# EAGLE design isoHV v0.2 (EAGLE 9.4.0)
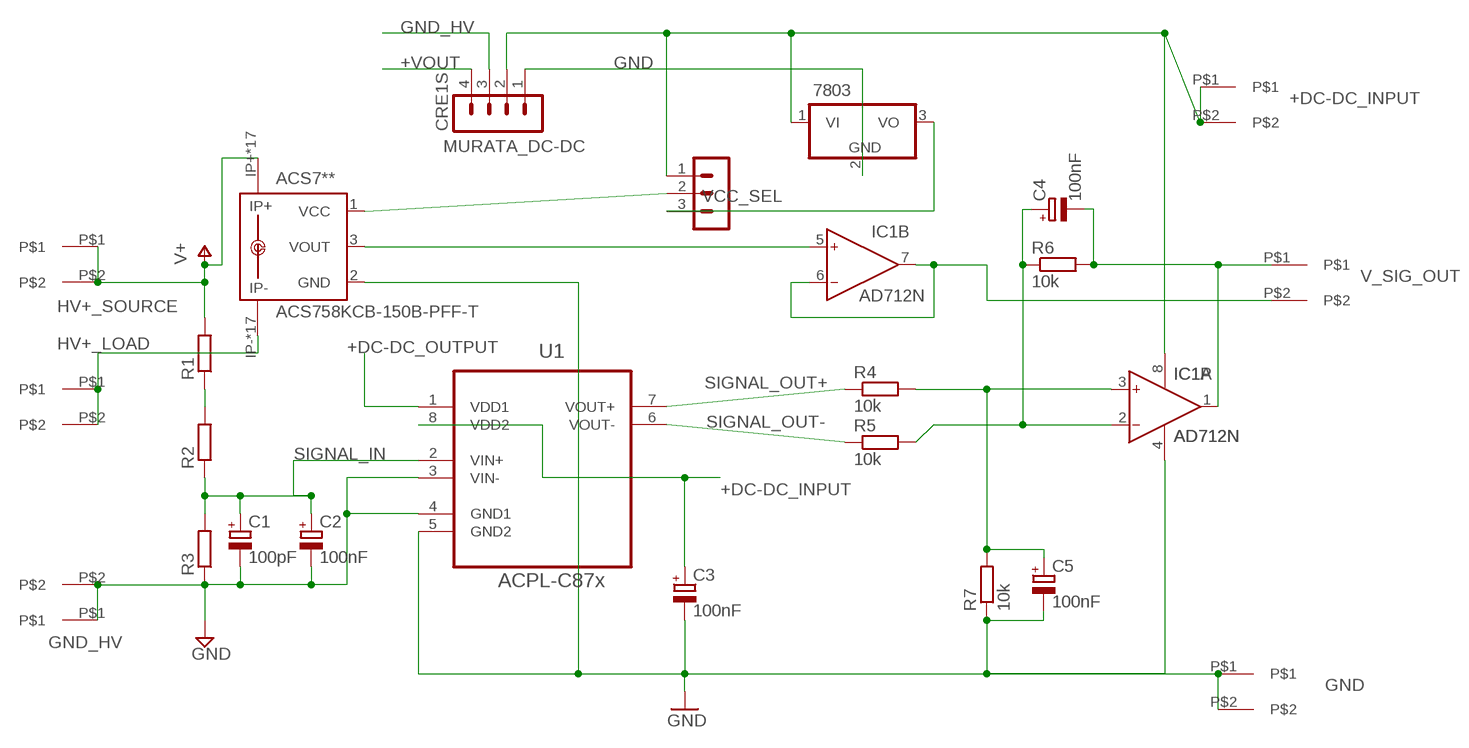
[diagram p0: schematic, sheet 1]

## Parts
7803  7805TV  [TO220V]
ACS7**  ACS758KCB-150B-PFF-T  [CB-PFF]
C1  100pF  CPOL-EUB45181A  [B45181A]
C2  100nF  CPOL-EUB45181A  [B45181A]
C3  100nF  CPOL-EUB45181A  [B45181A]
C4  100nF  CPOL-EUB45181A  [B45181A]
C5  100nF  CPOL-EUB45181A  [B45181A]
CRE1S  MURATA_DC-DC  [MA04-1]
IC1  AD712N  [DIL08]
R1  R-EU_0411/15  [0411/15]
R2  R-EU_0411/15  [0411/15]
R3  R-EU_0411/15  [0411/15]
R4  10k  R-EU_0204/7  [0204/7]
R5  10k  R-EU_0204/7  [0204/7]
R6  10k  R-EU_0204/7  [0204/7]
R7  10k  R-EU_0204/7  [0204/7]
U1  ACPL-C87x  ACPL-C79B-000E  [SOIC127P1150X330-8N]
U$1  7.62MM_TERMINAL_BLOCK  [7.62MM]
U$2  7.62MM_TERMINAL_BLOCK  [7.62MM]
U$3  7.62MM_TERMINAL_BLOCK  [7.62MM]
U$4  7.62MM_TERMINAL_BLOCK  [7.62MM]
U$5  7.62MM_TERMINAL_BLOCK  [7.62MM]
U$6  7.62MM_TERMINAL_BLOCK  [7.62MM]
VCC_SEL  MA03-1  [MA03-1]

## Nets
+DC-DC_INPUT: 7803.1(VI) C3.+ CRE1S.2 IC1.8(P:V+) U1.8(VDD2) U$3.P$1 U$3.P$2 VCC_SEL.1
+DC-DC_OUTPUT: U1.1(VDD1)
+VOUT: CRE1S.4
C_SIG_OUT: IC1.6(B:IN-) IC1.7(B:OUT) U$5.P$2
GND: 7803.2(GND) ACS7**.2(GND) C3.- C5.- CRE1S.1 IC1.4(P:V-) R7.1 U1.5(GND2) U$4.P$1 U$4.P$2
GND_HV: C1.- C2.- CRE1S.3 R3.1 U1.3(VIN-) U1.4(GND1) U$2.P$1 U$2.P$2 ; supply symbol labelled GND
HV+_LOAD: ACS7**.IP- ACS7**.IP-@2(IP-) ACS7**.IP-@3(IP-) ACS7**.IP-@4(IP-) ACS7**.IP-@5(IP-) ACS7**.IP-@6(IP-) ACS7**.IP-@7(IP-) ACS7**.IP-@8(IP-) ACS7**.IP-@9(IP-) ACS7**.IP-@10(IP-) ACS7**.IP-@11(IP-) ACS7**.IP-@12(IP-) ACS7**.IP-@13(IP-) ACS7**.IP-@14(IP-) ACS7**.IP-@15(IP-) ACS7**.IP-@16(IP-) ACS7**.IP-@17(IP-) U$6.P$1 U$6.P$2
HV+_SOURCE: ACS7**.IP+ ACS7**.IP+@2(IP+) ACS7**.IP+@3(IP+) ACS7**.IP+@4(IP+) ACS7**.IP+@5(IP+) ACS7**.IP+@6(IP+) ACS7**.IP+@7(IP+) ACS7**.IP+@8(IP+) ACS7**.IP+@9(IP+) ACS7**.IP+@10(IP+) ACS7**.IP+@11(IP+) ACS7**.IP+@12(IP+) ACS7**.IP+@13(IP+) ACS7**.IP+@14(IP+) ACS7**.IP+@15(IP+) ACS7**.IP+@16(IP+) ACS7**.IP+@17(IP+) R1.2 U$1.P$1 U$1.P$2 ; supply symbol labelled V+
N$1: C5.+ IC1.3(A:IN+) R4.2 R7.2
N$2: R1.1 R2.2
N$3: ACS7**.1(VCC) VCC_SEL.2
N$5: C4.+ IC1.2(A:IN-) R5.2 R6.1
N$6: ACS7**.3(VOUT) IC1.5(B:IN+)
N$7: 7803.3(VO) VCC_SEL.3
SIGNAL_IN: C1.+ C2.+ R2.1 R3.2 U1.2(VIN+)
SIGNAL_OUT+: R4.1 U1.7(VOUT+)
SIGNAL_OUT-: R5.1 U1.6(VOUT-)
V_SIG_OUT: C4.- IC1.1(A:OUT) R6.2 U$5.P$1

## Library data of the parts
7803 = linear:78*: Positive VOLTAGE REGULATOR Source: http://cache.national.com/ds/LM/LM78L05.pdf http://www.fairchildsemi.com/ds/LM/LM7805.pdf
ACS7** = allegro:ACS758*: Thermally Enhanced, Fully Integrated, Hall Effect-Based Linear Current Sensor with 100 micro Ohm Current Conductor display layer 49 Reference in BRD and place VIAs on circles Source: http://www.allegromicro.com/en/Products/Part_Numbers/0758/0758.pdf; MPN: ACS7**; OC_FARNELL: 1718995; OC_NEWARK: 04R7129
C1-C5 = rcl:CPOL-EU: POLARIZED CAPACITOR, European symbol; SPICEPREFIX: C
CRE1S = murata_dc-dc:MURATA_DC-DC; MPN: cre1s
IC1 = analog-devices:AD712: Dual Precision, Low Cost, High Speed BiFET Op Amp Source: http://www.analog.com/static/imported-files/data_sheets/AD712.pdf; MF: ALTERA CORPORATION; MPN: AD712JNZ; OC_FARNELL: 9604898; OC_NEWARK: 59K4554
R1-R7 = rcl:R-EU_: RESISTOR, European symbol; SPICEPREFIX: R
U1 = Avago_By_element14_Batch_1:ACPL-C79B-000E: Precision Miniature Isolation Amplifiers; DESCRIPTION: Precision Miniature Isolation Amplifiers; MPN: ACPL-C79B-000E; OC_FARNELL: 1854253; OC_NEWARK: 74R5803; PACKAGE: SOIC-8; SUPPLIER: AVAGO TECHNOLOGIES
U$1-U$6 = 7.62mm terminal block:7.62MM_TERMINAL_BLOCK
VCC_SEL = con-lstb:MA03-1: PIN HEADER; OC_FARNELL: unknown; OC_NEWARK: unknown

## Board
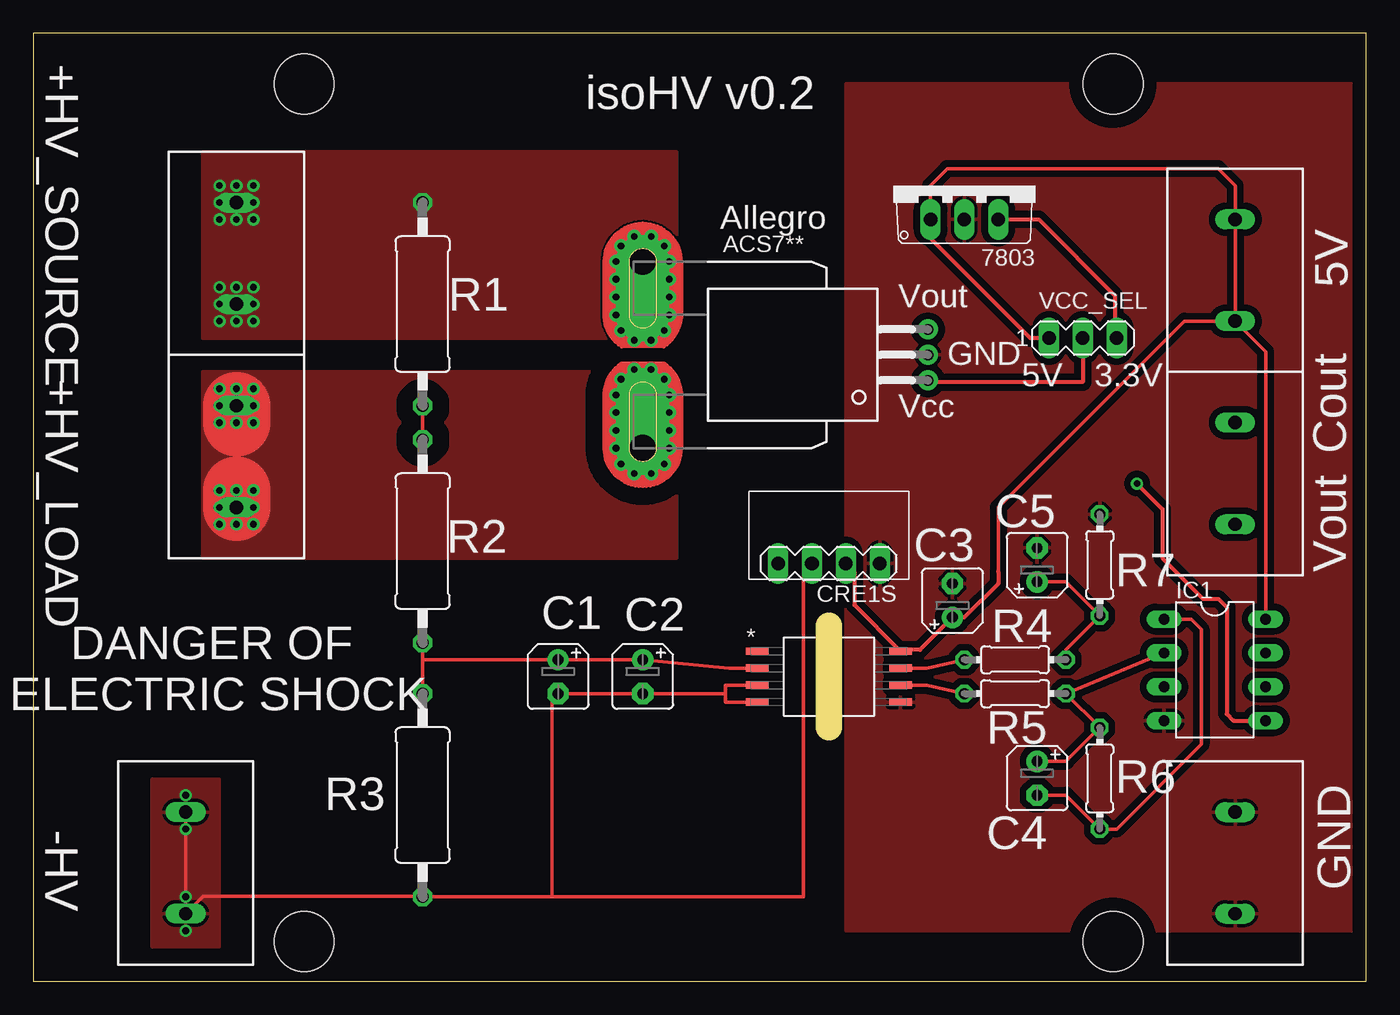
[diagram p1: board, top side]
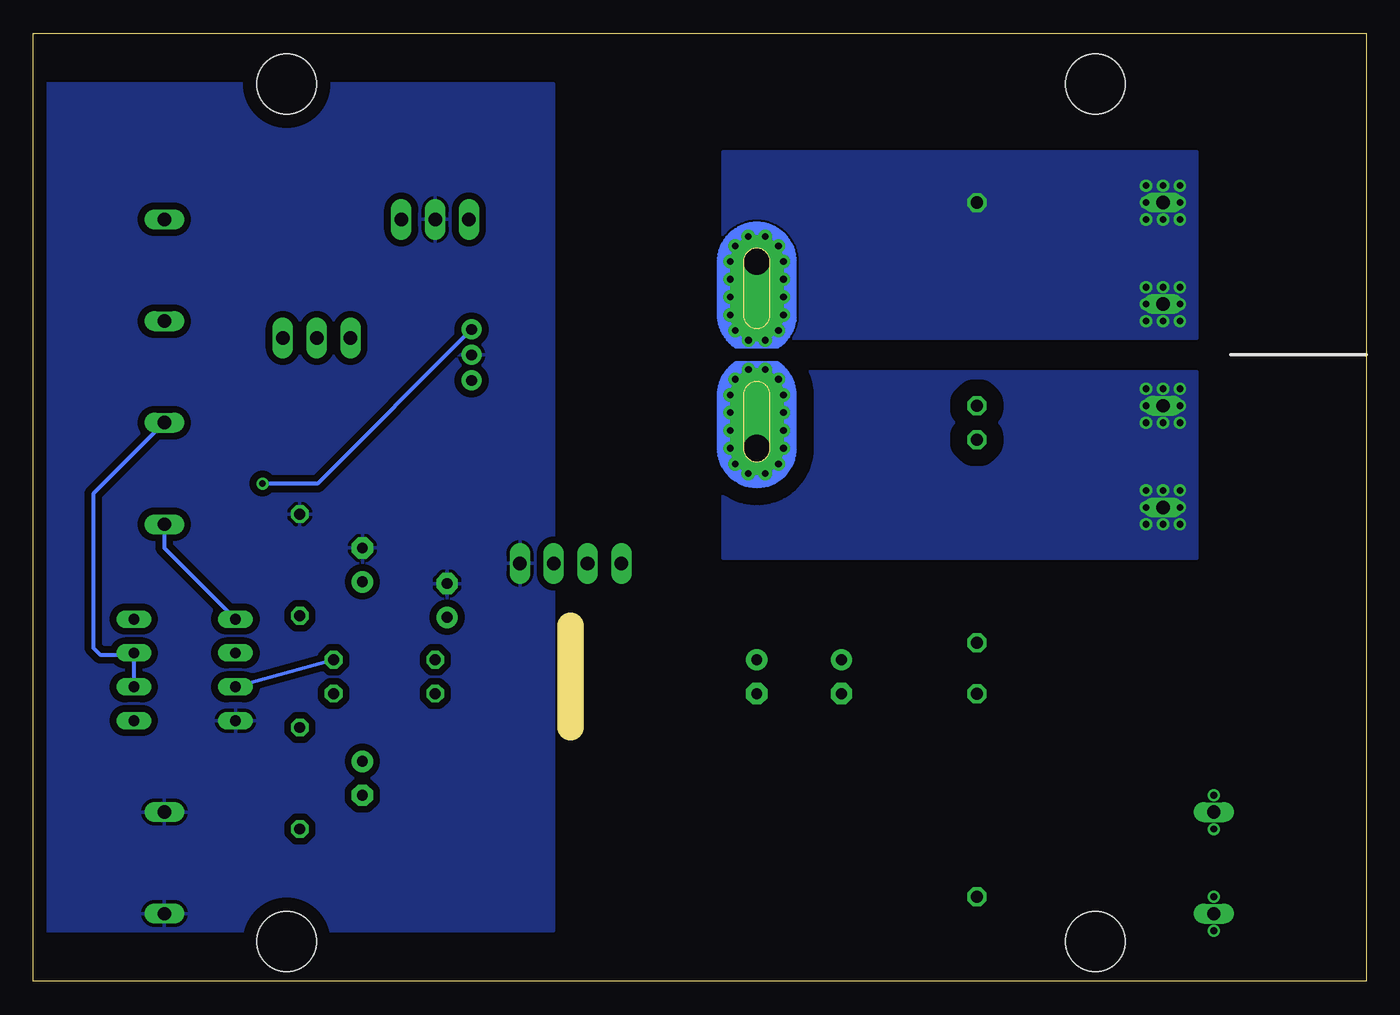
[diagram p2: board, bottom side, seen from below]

Size 100 x 71.11 mm. Coordinates in mm from the lower left corner, seen from the top.
Outline: 0,0 100,0 100,71.11 0,71.11 0,0
Copper layers (1*16): Top 0.035mm / dielectric 0.15mm / Bottom 0.035mm
Design rules "default *": minimum track width 10mil, minimum drill 0.35mm, track to track 6mil, track to pad 6mil, pad to pad 6mil, via to via 6mil, smd to smd 6mil, copper to edge 40mil, drill to drill 6mil, minimum pad ring 10mil, minimum via ring 8mil, stop-mask expansion 4mil, vias tented up to drill 0mil, thermal gap 10mil
Holes 4.5 mm at 20.32,67.31 20.32,3 81,3 81,67.31
Milling: 1 lines

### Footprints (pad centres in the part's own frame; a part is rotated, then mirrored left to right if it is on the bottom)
TO220V = drill 1.016 long: 1 -2.54,-2.54; 2 0,-2.54; 3 2.54,-2.54
CB-PFF = drill 0.8 pad 1.5: 1 -1.91,-21.4; 2 0,-21.4; 3 1.91,-21.4 | drill 2 pad 4 offset: IP+ 7,0; IP- -7,0 | drill 0.5 pad 0.9: IP+@2 8.89,0.635; IP+@3 8.89,-0.635; IP+@4 8.175,-1.625; IP+@5 7,-2; IP+@6 5.675,-2; IP+@7 4.35,-2; IP+@8 3,-2; IP+@9 1.825,-1.625; IP+@10 1.1,-0.625; IP+@11 1.1,0.625; IP+@12 1.825,1.625; IP+@13 3,2; IP+@14 4.35,2; IP+@15 5.675,2; IP+@16 7,2; IP+@17 8.175,1.625; IP-@2 -8.89,0.635; IP-@3 -8.89,-0.635; IP-@4 -8.175,-1.625; IP-@5 -7,-2; IP-@6 -5.675,-2; IP-@7 -4.325,-2; IP-@8 -3,-2; IP-@9 -1.825,-1.625; IP-@10 -1.1,-0.625; IP-@11 -1.1,0.625; IP-@12 -1.825,1.625; IP-@13 -3,2; IP-@14 -4.325,2; IP-@15 -5.675,2; IP-@16 -7,2; IP-@17 -8.175,1.625
B45181A = drill 0.813 pad 1.6: + -1.27,0 | drill 0.813 pad 1.6 octagon: - 1.27,0
MA04-1 = drill 1.016 long: 1 -3.81,0; 2 -1.27,0; 3 1.27,0; 4 3.81,0
DIL08 = drill 0.813 long: 1 -3.81,-3.81; 2 -1.27,-3.81; 3 1.27,-3.81; 4 3.81,-3.81; 5 3.81,3.81; 6 1.27,3.81; 7 -1.27,3.81; 8 -3.81,3.81
0411/15 = drill 0.914 octagon: 1 -7.62,0; 2 7.62,0
0204/7 = drill 0.813 octagon: 1 -3.81,0; 2 3.81,0
SOIC127P1150X330-8N = smd 1.702 x 0.559: 1 -5.385,1.905; 2 -5.385,0.635; 3 -5.385,-0.635; 4 -5.385,-1.905; 5 5.385,-1.905; 6 5.385,-0.635; 7 5.385,0.635; 8 5.385,1.905
7.62MM = drill 1 long: P$1 0,-3.81; P$2 0,3.81
MA03-1 = drill 1.016 long: 1 -2.54,0; 2 0,0; 3 2.54,0

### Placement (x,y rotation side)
7803  69.85,59.69 0 top
ACS7**  45.72,46.99 90 top
C1  39.37,22.86 270 top
C2  45.72,22.86 270 top
C3  68.96,28.57 90 top
C4  75.31,15.24 270 top
C5  75.31,31.24 90 top
CRE1S  59.69,31.35 180 top
IC1  88.65,23.37 270 top
R1  29.21,50.8 90 top
R2  29.21,33.02 90 top
R3  29.21,13.97 90 top
R4  73.66,24.13 0 top
R5  73.66,21.59 0 top
R6  80.01,15.24 270 top
R7  80.01,31.24 270 top
U1  59.69,22.86 0 top
U$1  15.24,54.61 180 top
U$2  11.43,8.89 0 top
U$3  90.17,53.34 0 top
U$4  90.17,8.89 180 top
U$5  90.17,38.1 0 top
U$6  15.24,39.37 0 top
VCC_SEL  78.74,48.26 0 top

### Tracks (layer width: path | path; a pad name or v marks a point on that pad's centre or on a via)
+DC-DC_INPUT
  Top 0.254: 65.08,24.88 U1.8 | IC1.8 92.46,47.24 U$3.P$1 | U$3.P$1 U$3.P$2 90.17,59.69 88.9,60.96 68.58,60.96 67.31,59.69 7803.1 | 72.39,30.73 72.39,35.56 86.36,49.53 U$3.P$1
  Top 0.305: 7803.1 67.31,55.75 74.8,48.26 VCC_SEL.1 | 72.39,30.73 72.39,29.84 69.85,27.3 C3.+ 66.53,24.88 65.08,24.88 | U1.8 61.59,28.25 61.59,30.71 CRE1S.2
C_SIG_OUT
  Bottom 0.305: U$5.P$2 95.5,36.58 95.5,25.02 95,24.51 92.58,24.51 IC1.7 IC1.6
GND
  pour Bottom (isolate 0.508): 100.33,67.31 100.33,3.81 60.96,3.81 60.96,67.31
  pour Top (isolate 0.508): 60.96,67.31 60.96,3.81 100.33,3.81 100.33,67.31
GND_HV  (via drill 0.5)
  Top 0.254: U1.3 51.94,22.23 51.94,21.59 | 51.94,21.59 51.94,20.95 U1.4 | U$2.P$2 v11.43,11.43 v11.43,6.35 U$2.P$1 12.74,6.39 29.17,6.39 R3.1 | R3.1 38.9,6.35 38.9,21.12 C1.- C2.- 51.94,21.59 | R3.1 57.78,6.35 57.78,30.71 CRE1S.3
  other vias: 11.43,13.97 11.43,3.81
  pour Top: 8.89,15.24 13.97,15.24 13.97,2.54 8.89,2.54
HV+_LOAD  (via drill 0.5)
  Top 5.08: U$6.P$1 v15.24,36.83 | v15.24,41.91 U$6.P$2
  other vias: 13.97,44.45 15.24,44.45 16.51,44.45 16.51,43.18 16.51,41.91 13.97,41.91 13.97,43.18 16.51,36.83 16.51,35.56 16.51,34.29 15.24,34.29 13.97,34.29 13.97,35.56 13.97,36.83
  pour Top (isolate 1.27, no thermals): 46.99,31.75 12.7,31.75 12.7,45.72 48.26,45.72 48.26,31.75
  pour Bottom (isolate 1.27, no thermals): 46.99,45.72 12.7,45.72 12.7,31.75 48.26,31.75 48.26,45.72
HV+_SOURCE  (via drill 0.5)
  other vias: 13.97,52.07 15.24,52.07 16.51,52.07 16.51,50.8 16.51,49.53 15.24,49.53 13.97,49.53 13.97,50.8 15.24,57.15 16.51,57.15 16.51,58.42 16.51,59.69 15.24,59.69 13.97,59.69 13.97,58.42 13.97,57.15
  pour Top (no thermals): 46.99,48.26 12.7,48.26 12.7,62.23 48.26,62.23 48.26,48.26
  pour Bottom (no thermals): 13.97,48.26 48.26,48.26 48.26,62.23 12.7,62.23 12.7,48.26
N$1
  Top 0.254: R4.2 77.47,24.89 R7.2 77.47,29.97 C5.+
  Bottom 0.254: R4.2 IC1.3
N$2
  Top 0.254: R1.1 R2.2
N$3
  Top 0.305: VCC_SEL.2 78.74,44.96 67.24,44.96 ACS7**.1
N$5
  Top 0.254: IC1.2 R5.2 R6.1 77.47,16.51 C4.+
N$6  (via drill 0.5)
  Top 0.305: v82.8,37.34 84.71,35.43 84.71,31.75 87.76,28.7 88.9,28.7 89.53,28.07 89.53,20.07 90.04,19.56 IC1.5
  Bottom 0.305: ACS7**.3 78.68,37.34 v82.8,37.34
N$7
  Top 0.305: 7803.3 75.44,57.15 81.15,51.44 81.15,48.39 VCC_SEL.3
SIGNAL_IN
  Top 0.254: R2.1 R3.2 29.21,24.13 C1.+ C2.+ 52.2,23.5 U1.2
SIGNAL_OUT+
  Top 0.254: U1.7 67.06,23.5 R4.1
SIGNAL_OUT-
  Top 0.254: U1.6 67.06,22.23 R5.1
V_SIG_OUT
  Top 0.254: C4.- 77.47,13.97 R6.2 81.28,11.43 87.63,17.78 87.63,26.42 86.87,27.18 IC1.1
  Bottom 0.305: U$5.P$1 90.17,32.51 IC1.1

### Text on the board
tNames: +HV_SOURCE | isoHV v0.2 | Allegro | 5V | Vout | GND | 5V | 3.3V | +HV_LOAD | Vcc | Cout | Vout | DANGER OF / ELECTRIC SHOCK | -HV | GND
